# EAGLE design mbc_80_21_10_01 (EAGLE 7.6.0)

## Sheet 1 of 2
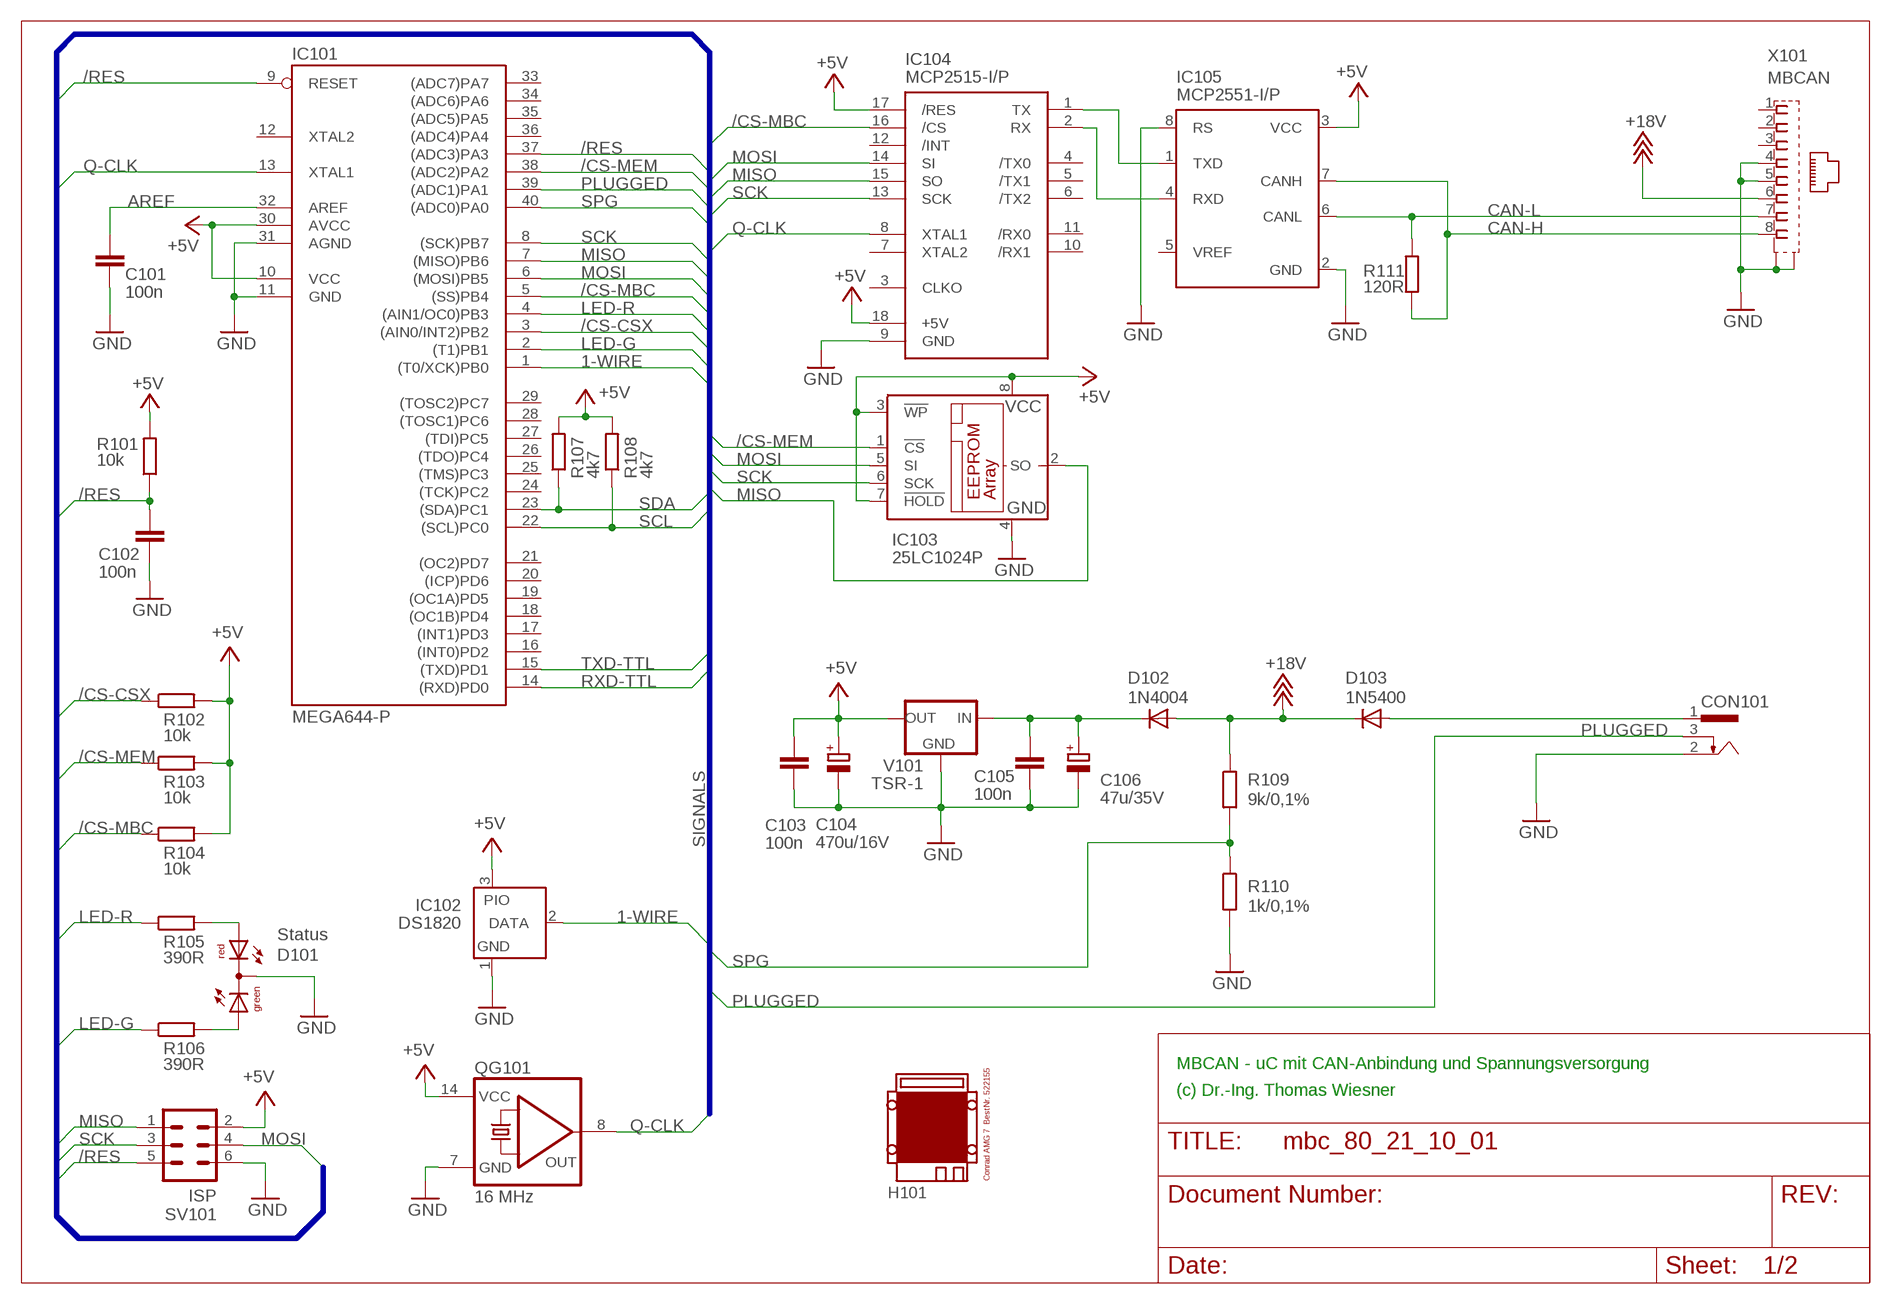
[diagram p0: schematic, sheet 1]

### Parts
C101  100n  C-EU025-025X050  [C025-025X050]
C102  100n  C-EU025-025X050  [C025-025X050]
C103  100n  C-EU025-025X050  [C025-025X050]
C104  470u/16V  CPOL-EUE3.5-8  [E3,5-8]
C105  100n  C-EU025-025X050  [C025-025X050]
C106  47u/35V  CPOL-EUE2.5-7  [E2,5-7]
CON101  POWER-JACK  [POWER-JACK]
D101  Status  DUOLED5MM  [DUOLED5MM]
D102  1N4004  [DO41-10]
D103  1N5400  [DO201-15]
H101  MODULGEHÄUSE-AMG-7  [MODULGEHÄUSE-AMG-7]
IC101  MEGA644-P  MEGA323-P  [DIL40]
IC102  DS1820  DS2405  [TO92-]
IC103  25LC1024P  25LC040P  [DIL8]
IC104  MCP2515-I/P  MCP2510-I/P  [DIL18]
IC105  MCP2551-I/P  PCA82C250  [DIL08]
QG101  16 MHz  QG5860  [DIL14S]
R101  10k  R-EU_0207/10  [0207/10]
R102  10k  R-EU_0207/10  [0207/10]
R103  10k  R-EU_0207/10  [0207/10]
R104  10k  R-EU_0207/10  [0207/10]
R105  390R  R-EU_0207/10  [0207/10]
R106  390R  R-EU_0207/10  [0207/10]
R107  4k7  R-EU_0207/10  [0207/10]
R108  4k7  R-EU_0207/10  [0207/10]
R109  9k/0,1%  R-EU_0207/10  [0207/10]
R110  1k/0,1%  R-EU_0207/10  [0207/10]
R111  120R  R-EU_0207/10  [0207/10]
SV101  ISP  ML6  [ML6]
V101  TSR-1  [TRACO-TSR-1]
X101  MBCAN  0446200002  [0446200002]

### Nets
1-WIRE: IC101.1((T0/XCK)PB0) IC102.2(DATA)
+5V: C103.1 C104.+ IC101.10(VCC) IC101.30(AVCC) IC102.3(PIO) IC103.3(!WP) IC103.7(!HOLD) IC103.8(VCC) IC104.17(/RES) IC104.18(+5V) IC105.3(VCC) QG101.14(VCC) R101.2 R102.2 R103.2 R104.2 R107.2 R108.2 SV101.2 V101.OUT ; also sheet 2
+18V: D102.A D103.C R109.1 X101.6
/CS-CSX: IC101.3((AIN0/INT2)PB2) R102.1 ; also sheet 2
/CS-MBC: IC101.5((SS)PB4) IC104.16(/CS) R104.1
/CS-MEM: IC101.38((ADC2)PA2) IC103.1(!CS) R103.1
/RES: C102.1 IC101.9(RESET) IC101.37((ADC3)PA3) R101.1 SV101.5
AREF: C101.1 IC101.32(AREF)
CAN-H: IC105.7(CANH) R111.1 X101.8
CAN-L: IC105.6(CANL) R111.2 X101.7
GND: C101.2 C102.2 C103.2 C104.- C105.2 C106.- CON101.2 D101.K(C) IC101.11(GND) IC101.31(AGND) IC102.1(GND) IC103.4(GND) IC104.9(GND) IC105.2(GND) IC105.8(RS) QG101.7(GND) R110.2 SV101.6 V101.GND X101.4 X101.5 X101.S@1(S1) X101.S@2(S2) ; also sheet 2
LED-G: IC101.2((T1)PB1) R106.1
LED-R: IC101.4((AIN1/OC0)PB3) R105.1
MISO: IC101.7((MISO)PB6) IC103.2(SO) IC104.15(SO) SV101.1 ; also sheet 2
MOSI: IC101.6((MOSI)PB5) IC103.5(SI) IC104.14(SI) SV101.4 ; also sheet 2
N$1: IC104.1(TX) IC105.1(TXD)
N$2: IC104.2(RX) IC105.4(RXD)
N$6: C105.1 C106.+ D102.C V101.IN
N$9: D101.AR R105.2
N$13: D101.AG R106.2
PLUGGED: CON101.3 IC101.39((ADC1)PA1)
Q-CLK: IC101.13(XTAL1) IC104.8(XTAL1) QG101.8(OUT) ; also sheet 2
RXD-TTL: IC101.14((RXD)PD0) ; also sheet 2
SCK: IC101.8((SCK)PB7) IC103.6(SCK) IC104.13(SCK) SV101.3 ; also sheet 2
SCL: IC101.22((SCL)PC0) R108.1 ; also sheet 2
SDA: IC101.23((SDA)PC1) R107.1 ; also sheet 2
SPG: IC101.40((ADC0)PA0) R109.2 R110.1
TXD-TTL: IC101.15((TXD)PD1) ; also sheet 2
V-NETZTEIL: CON101.1 D103.A
Unconnected: IC101.12(XTAL2) IC101.16((INT0)PD2) IC101.17((INT1)PD3) IC101.18((OC1B)PD4) IC101.19((OC1A)PD5) IC101.20((ICP)PD6) IC101.21((OC2)PD7) IC101.24((TCK)PC2) IC101.25((TMS)PC3) IC101.26((TDO)PC4) IC101.27((TDI)PC5) IC101.28((TOSC1)PC6) IC101.29((TOSC2)PC7) IC101.33((ADC7)PA7) IC101.34((ADC6)PA6) IC101.35((ADC5)PA5) IC101.36((ADC4)PA4) IC104.3(CLKO) IC104.4(/TX0) IC104.5(/TX1) IC104.6(/TX2) IC104.7(XTAL2) IC104.10(/RX1) IC104.11(/RX0) IC104.12(/INT) IC105.5(VREF) X101.1 X101.2 X101.3

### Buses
SIGNALS

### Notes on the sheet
- MBCAN - uC mit CAN-Anbindung und Spannungsversorgung
- (c) Dr.-Ing. Thomas Wiesner

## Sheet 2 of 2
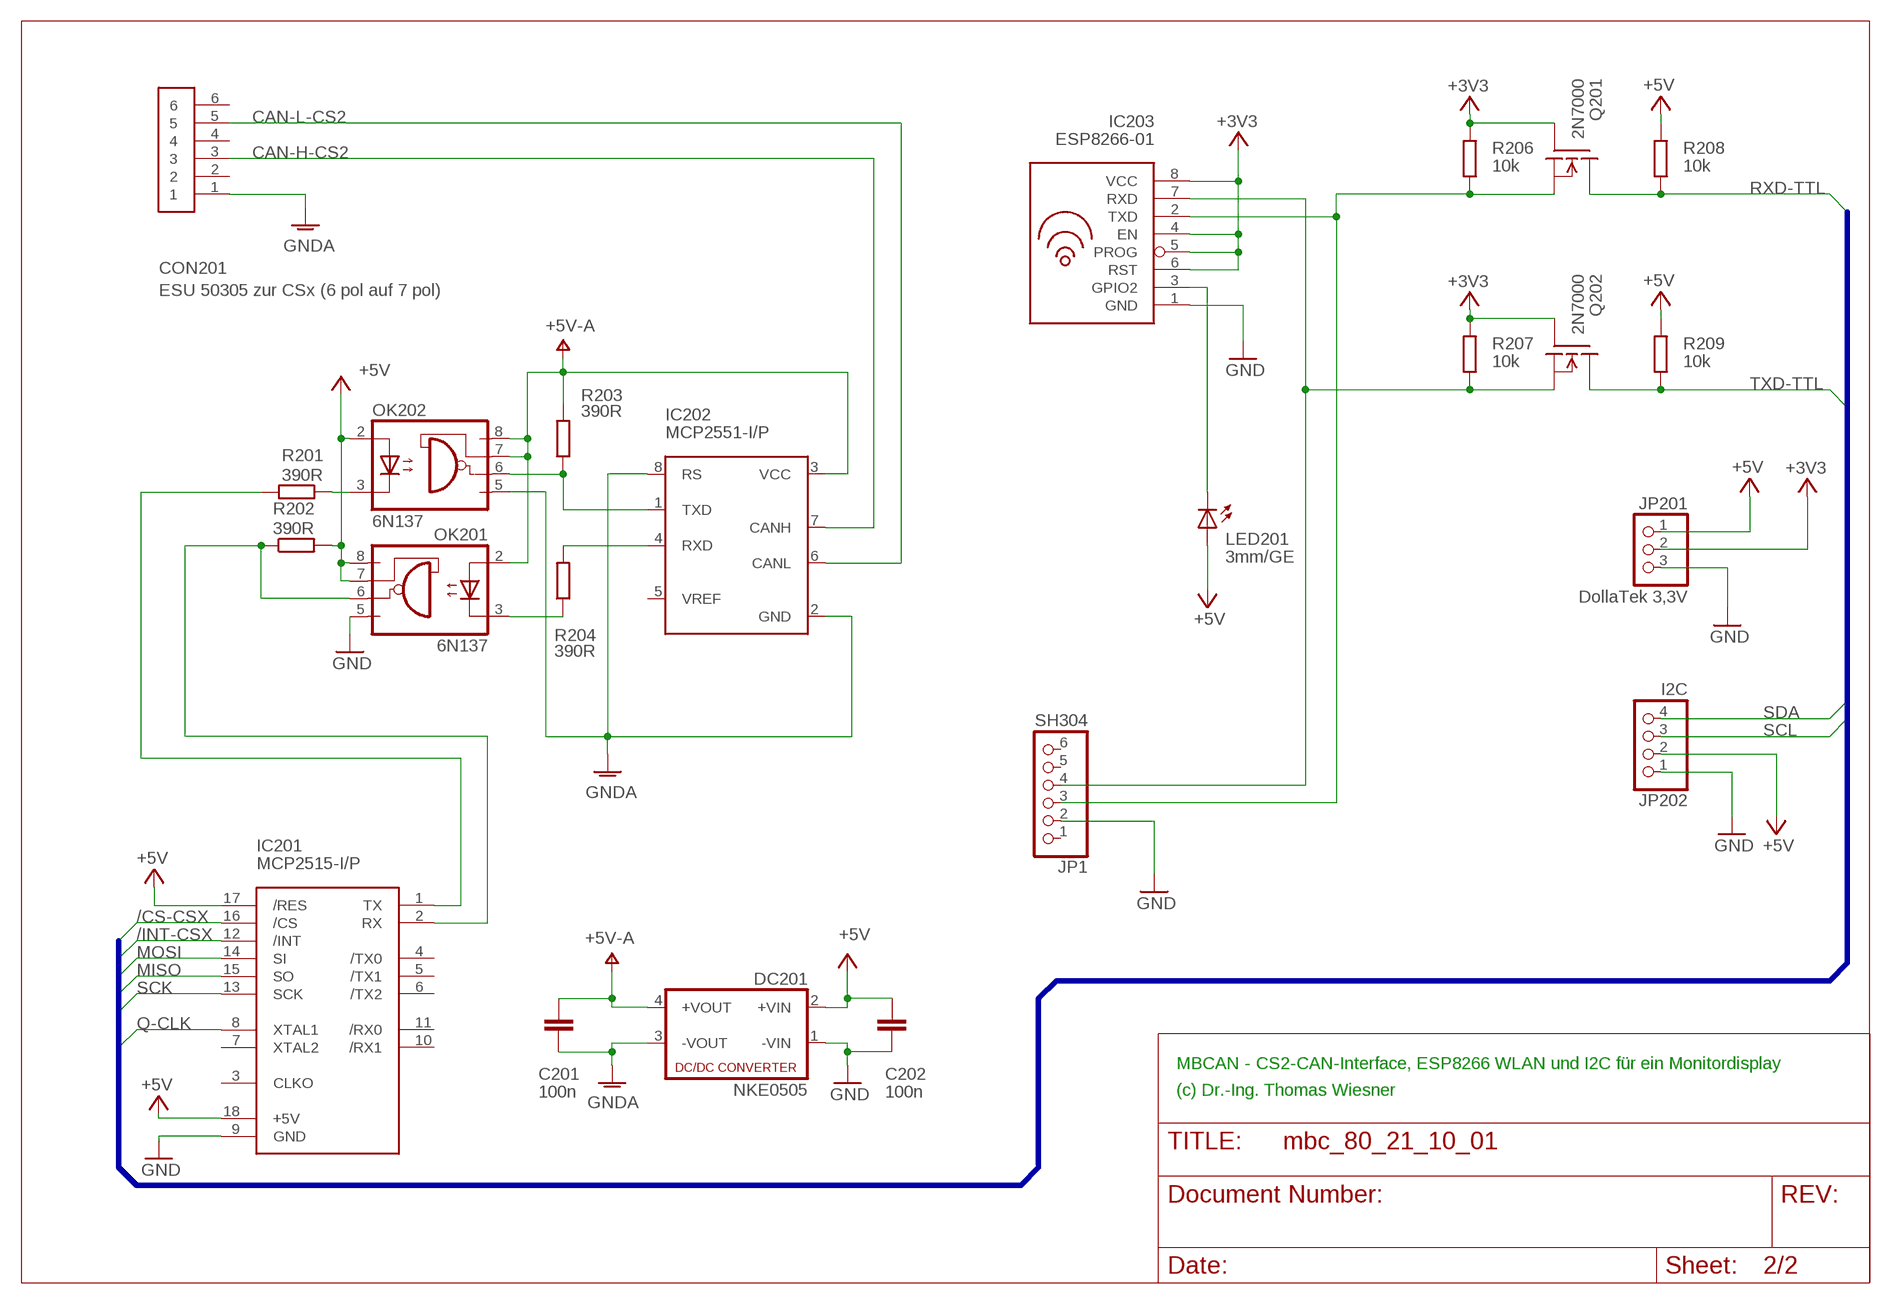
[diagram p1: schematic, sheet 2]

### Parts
C201  100n  C-EU025-025X050  [C025-025X050]
C202  100n  C-EU025-025X050  [C025-025X050]
CON201  ESU 50305 zur CSx (6 pol auf 7 pol)  TM-0508-A6  [MINI-DIN-6-POL]
DC201  NKE0505  NME  [NME]
IC201  MCP2515-I/P  MCP2510-I/P  [DIL18]
IC202  MCP2551-I/P  PCA82C250  [DIL08]
IC203  ESP8266-01  [ESP8266-01]
JP1  SH304  PINHD-1X6  [1X06]
JP201  DollaTek 3,3V  PINHD-1X3  [1X03]
JP202  I2C  PINHD-1X4  [1X04]
LED201  3mm/GE  LED3MM  [LED3MM]
OK201  6N137  [DIL08]
OK202  6N137  [DIL08]
Q201  2N7000  TN0602N3  [TO-92]
Q202  2N7000  TN0602N3  [TO-92]
R201  390R  R-EU_0207/10  [0207/10]
R202  390R  R-EU_0207/10  [0207/10]
R203  390R  R-EU_0207/10  [0207/10]
R204  390R  R-EU_0207/10  [0207/10]
R206  10k  R-EU_0207/10  [0207/10]
R207  10k  R-EU_0207/10  [0207/10]
R208  10k  R-EU_0207/10  [0207/10]
R209  10k  R-EU_0207/10  [0207/10]

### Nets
+3V3: IC203.4(EN) IC203.5(PROG) IC203.6(RST) IC203.8(VCC) JP201.2 Q201.2(G) Q202.2(G) R206.2 R207.2
+5V: C202.1 DC201.2(+VIN) IC201.17(/RES) IC201.18(+5V) JP201.1 JP202.2 LED201.A OK201.7(VE) OK201.8(VCC) OK202.2(A) R202.2 R208.2 R209.2 ; also sheet 1
+5V-A: C201.1 DC201.4(+VOUT) IC202.3(VCC) OK201.2(A) OK202.7(VE) OK202.8(VCC) R203.2
/CS-CSX: IC201.16(/CS) ; also sheet 1
/INT-CSX: IC201.12(/INT)
CAN-H-CS2: CON201.3 IC202.7(CANH)
CAN-L-CS2: CON201.5 IC202.6(CANL)
GND: C202.2 DC201.1(-VIN) IC201.9(GND) IC203.1(GND) JP1.2 JP201.3 JP202.1 OK201.5(GND) ; also sheet 1
GNDA: C201.2 CON201.1 DC201.3(-VOUT) IC202.2(GND) IC202.8(RS) OK202.5(GND)
MISO: IC201.15(SO) ; also sheet 1
MOSI: IC201.14(SI) ; also sheet 1
N$3: IC203.3(GPIO2) LED201.K(C)
N$5: IC203.2(TXD) JP1.3 Q201.1(S) R206.1
N$8: IC203.7(RXD) JP1.4 Q202.1(S) R207.1
N$10: IC201.1(TX) R201.2
N$40: IC202.1(TXD) OK202.6(VO) R203.1
N$43: OK201.3(C) R204.1
N$44: IC202.4(RXD) R204.2
N$46: OK202.3(C) R201.1
N$48: IC201.2(RX) OK201.6(VO) R202.1
Q-CLK: IC201.8(XTAL1) ; also sheet 1
RXD-TTL: Q201.3(D) R208.1 ; also sheet 1
SCK: IC201.13(SCK) ; also sheet 1
SCL: JP202.3 ; also sheet 1
SDA: JP202.4 ; also sheet 1
TXD-TTL: Q202.3(D) R209.1 ; also sheet 1
Unconnected: CON201.2 CON201.4 CON201.6 IC201.3(CLKO) IC201.4(/TX0) IC201.5(/TX1) IC201.6(/TX2) IC201.7(XTAL2) IC201.10(/RX1) IC201.11(/RX0) IC202.5(VREF) JP1.1 JP1.5 JP1.6

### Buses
SIGNALS

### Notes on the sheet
- MBCAN - CS2-CAN-Interface, ESP8266 WLAN und I2C für ein Monitordisplay
- (c) Dr.-Ing. Thomas Wiesner

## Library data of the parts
C101-C103 C105 C201 C202 = rcl:C-EU: CAPACITOR, European symbol
C104 C106 = rcl:CPOL-EU: POLARIZED CAPACITOR, European symbol
CON101 = mbc:POWER-JACK
CON201 = mbc:TM-0508-A6: MINI-DIN 6-pol Printbuchse Reichelt Bestellnummer EB-DIO M06
D101 = led:DUOLED5MM: DUO LED 2 colors, 5 mm, round
D102 = diode:1N4004: DIODE
D103 = diode:1N5400: DIODE
DC201 = dc-dc-converter:NME: DC-DC CONVERTER; MF: C & D TECHNOLOGIES, INC; MPN: NME1205D; OC_FARNELL: 1021466; OC_NEWARK: 98B8198
H101 = mbc:MODULGEHÄUSE-AMG-7: Gehäuse
IC101 = atmel:MEGA323-P: MICROCONTROLLER 32 Kbytes FLASH 2 Kbytes SRAM 1 Kbytes EEPROM USART 8-channel 10 bit ADC Source: avr.lbr; OC_FARNELL: unknown; OC_NEWARK: unknown
IC102 = maxim:DS2405: Addressable Switch DALLAS Semiconductor; MF: DALLAS SEMICONDUCTOR; MPN: DS2405; OC_FARNELL: 1188025; OC_NEWARK: 06F4645
IC103 = microchip:25*: Serial EEPROM 4K/ 8K , SPI bus; MF: MICROCHIP; MPN: 25LC040/P; OC_FARNELL: 9758100; OC_NEWARK: 96K4091
IC104 IC201 = mbc:MCP2510: BASIC-CAN 2.0a Controller Stand-alone CAN controller von Microchip
IC105 IC202 = micro-philips:PCA82C250: CAN CONTROLLER INTERFACE; OC_FARNELL: 3692358; OC_NEWARK: unknown
IC203 = mbc:ESP8266-01
JP1 = pinhead:PINHD-1X6: PIN HEADER
JP201 = pinhead:PINHD-1X3: PIN HEADER
JP202 = pinhead:PINHD-1X4: PIN HEADER
LED201 = led:LED: LED
OK201 OK202 = optocoupler:6N137: MOTOROLA OPTO COUPLER; MPN: 6N137; OC_FARNELL: 1328376; OC_NEWARK: 52M1895
Q201 Q202 = transistor-fet:TN0602N3: N-Channel Enhancement MOSFET 20V; 4A; 0,75Ohm
QG101 = crystal:QG5860: CRYSTAL RESONATOR; OC_FARNELL: unknown; OC_NEWARK: unknown
R101-R111 R201-R204 R206-R209 = resistor:R-EU_: RESISTOR, European symbol
SV101 = con-ml:ML6: HARTING; OC_FARNELL: unknown; OC_NEWARK: unknown
V101 = mbc:TSR-1: Spannungsregler Hersteller: TRACO Typ: TSR-1 5V: TSR 1-2450 Spg: 5V Strom: 1A Reichelt TSR 1-2450
X101 = mbc:0446200002: RJ-45 INVERTED MODULAR JACK ASSEMBLY WITH RJ-11 KEEPOUT FEATURE Source: Data sheet MOLEX 0446200002 BUCHSE, RJ45, GESCHIRMT Source: Farnell; MF: MOLEX; MPN: 0446200002; OC_FARNELL: 9251910

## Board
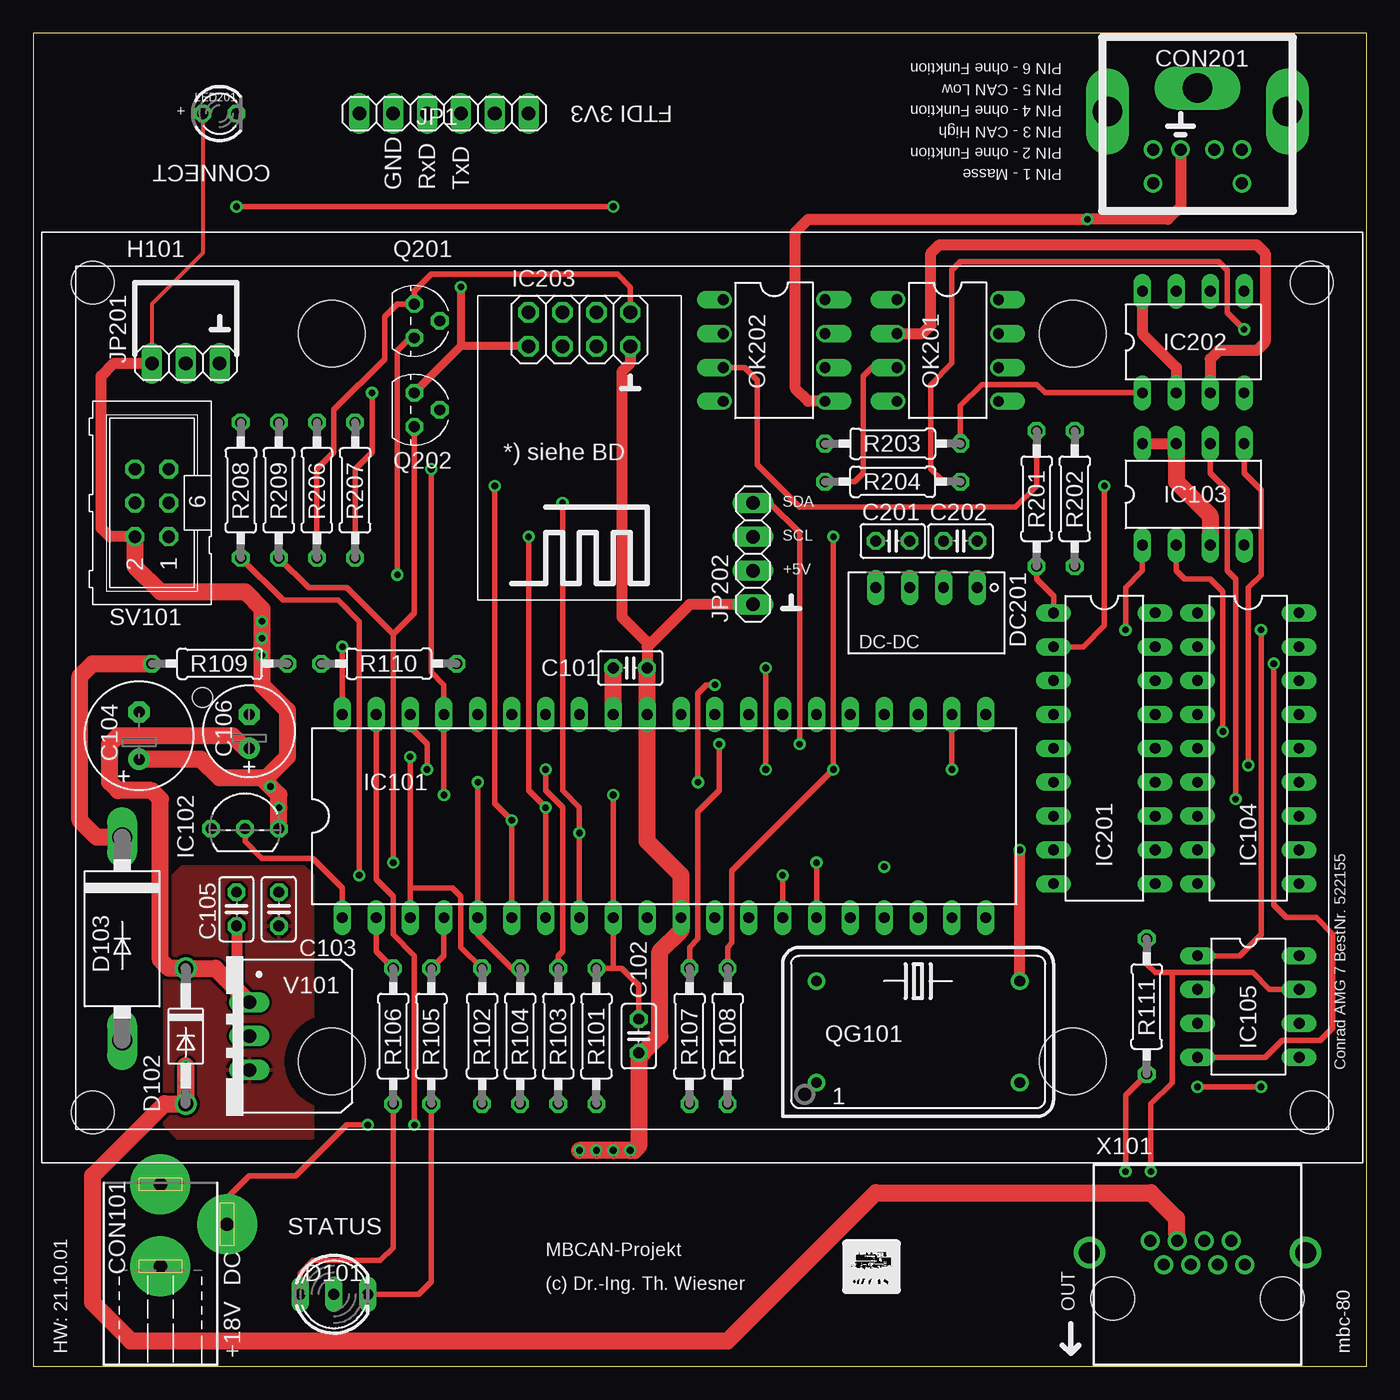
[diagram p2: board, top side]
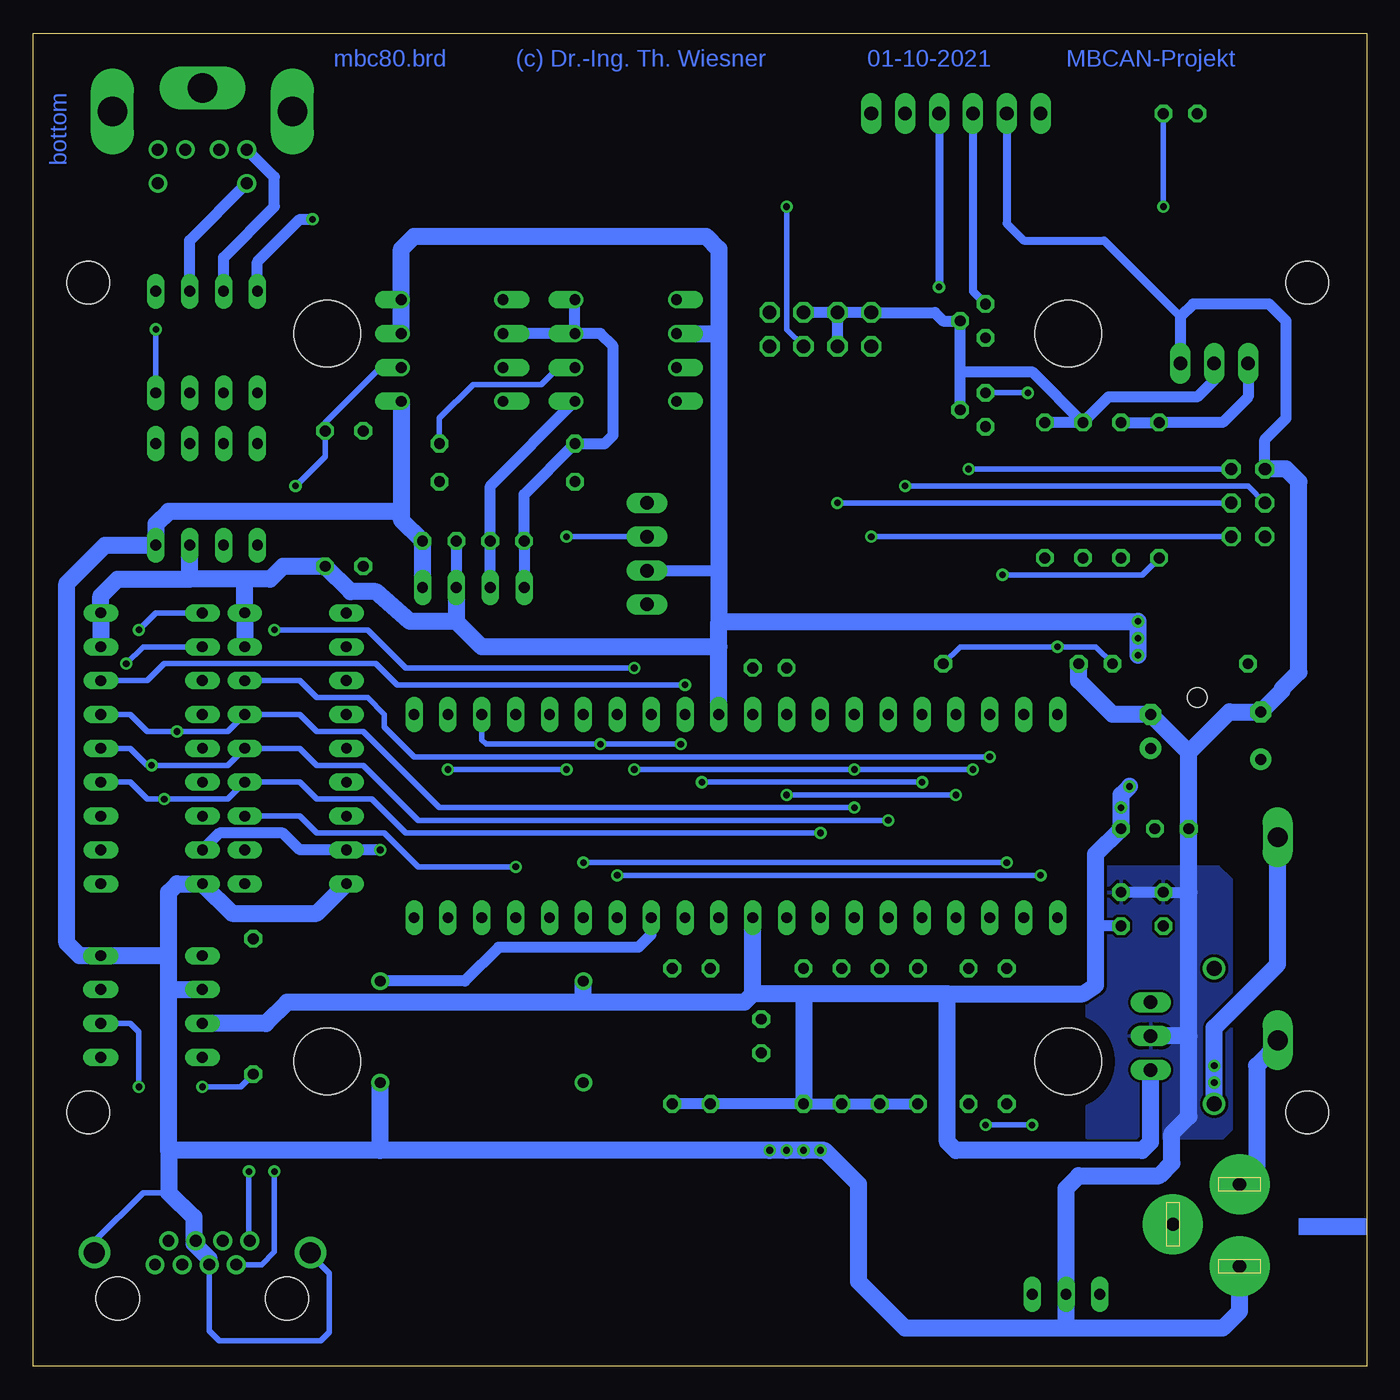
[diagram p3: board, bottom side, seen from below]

Size 99.99 x 100 mm. Coordinates in mm from the lower left corner, seen from the top.
Outline: 0,0 99.99,0 99.99,100 0,100 0,0
Copper layers (1*16): Top 0.035mm / dielectric 1.5mm / Bottom 0.035mm
Design rules "default *": minimum track width 10mil, minimum drill 0.5mm, track to track 8mil, track to pad 8mil, pad to pad 8mil, via to via 8mil, smd to smd 8mil, copper to edge 40mil, drill to drill 8mil, minimum pad ring 10mil, minimum via ring 8mil, stop-mask expansion 4mil, vias tented up to drill 0mil, thermal gap 10mil

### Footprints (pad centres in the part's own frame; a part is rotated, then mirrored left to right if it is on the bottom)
C025-025X050 = drill 0.813 octagon: 1 -1.27,0; 2 1.27,0
E3,5-8 = drill 0.813 pad 1.6: + -1.778,0 | drill 0.813 pad 1.6 octagon: - 1.778,0
E2,5-7 = drill 0.813 pad 1.6: + -1.27,0 | drill 0.813 pad 1.6 octagon: - 1.27,0
POWER-JACK = drill 1 pad 4.5: 1 0,6.03; 2 0,-0.12; 3 5,3.03
MINI-DIN-6-POL = drill 0.9: 1 -1.27,-4.604; 2 1.27,-4.604; 3 -3.334,-4.604; 4 3.334,-4.604; 5 -3.334,-7.144; 6 3.334,-7.144 | drill 2.2 pad 2.54 long: A1 0,0.01; A2 -6.75,-1.746; A3 6.75,-1.746
DUOLED5MM = drill 0.813 long: AG -2.54,0; AR 2.54,0; K 0,0
DO41-10 = drill 1.118: A 5.08,0; C -5.08,0
DO201-15 = drill 1.499 long: A 7.62,0; C -7.62,0
NME = drill 0.813 long: 1 0,3.81; 2 0,1.27; 3 0,-1.27; 4 0,-3.81
MODULGEHÄUSE-AMG-7 = hole 3.2: -45.72,-31.115; -45.72,31.115; 45.72,31.115; 45.72,-31.115 | hole 5: -27.781,-27.305; 27.781,-27.305; -27.781,27.305; 27.781,27.305 | hole 1.5: -37.465,0
DIL40 = drill 0.813 long: 1 -24.13,-7.62; 2 -21.59,-7.62; 3 -19.05,-7.62; 4 -16.51,-7.62; 5 -13.97,-7.62; 6 -11.43,-7.62; 7 -8.89,-7.62; 8 -6.35,-7.62; 9 -3.81,-7.62; 10 -1.27,-7.62; 11 1.27,-7.62; 12 3.81,-7.62; 13 6.35,-7.62; 14 8.89,-7.62; 15 11.43,-7.62; 16 13.97,-7.62; 17 16.51,-7.62; 18 19.05,-7.62; 19 21.59,-7.62; 20 24.13,-7.62; 21 24.13,7.62; 22 21.59,7.62; 23 19.05,7.62; 24 16.51,7.62; 25 13.97,7.62; 26 11.43,7.62; 27 8.89,7.62; 28 6.35,7.62; 29 3.81,7.62; 30 1.27,7.62; 31 -1.27,7.62; 32 -3.81,7.62; 33 -6.35,7.62; 34 -8.89,7.62; 35 -11.43,7.62; 36 -13.97,7.62; 37 -16.51,7.62; 38 -19.05,7.62; 39 -21.59,7.62; 40 -24.13,7.62
TO92- = drill 0.813 octagon: 1 -2.54,0; 2 0,0; 3 2.54,0
DIL8 = drill 0.813 long: 1 -3.81,-3.81; 2 -1.27,-3.81; 3 1.27,-3.81; 4 3.81,-3.81; 5 3.81,3.81; 6 1.27,3.81; 7 -1.27,3.81; 8 -3.81,3.81
DIL18 = drill 0.813 long: 1 -10.16,-3.81; 2 -7.62,-3.81; 3 -5.08,-3.81; 4 -2.54,-3.81 | drill 0.8 long: 5 0,-3.81; 6 2.54,-3.81; 7 5.08,-3.81; 8 7.62,-3.81; 9 10.16,-3.81; 10 10.16,3.81; 11 7.62,3.81; 12 5.08,3.81; 13 2.54,3.81; 14 0,3.81; 15 -2.54,3.81; 16 -5.08,3.81; 17 -7.62,3.81; 18 -10.16,3.81
DIL08 = drill 0.813 long: 1 -3.81,-3.81; 2 -1.27,-3.81; 3 1.27,-3.81; 4 3.81,-3.81; 5 3.81,3.81; 6 1.27,3.81; 7 -1.27,3.81; 8 -3.81,3.81
ESP8266-01 = drill 1.016 octagon: 1 3.81,-1.27; 2 3.81,1.27; 3 1.27,-1.27; 4 1.27,1.27; 5 -1.27,-1.27; 6 -1.27,1.27; 7 -3.81,-1.27; 8 -3.81,1.27
1X06 = drill 1.016 long: 1 -6.35,0; 2 -3.81,0; 3 -1.27,0; 4 1.27,0; 5 3.81,0; 6 6.35,0
1X03 = drill 1.016 long: 1 -2.54,0; 2 0,0; 3 2.54,0
1X04 = drill 1.016 long: 1 -3.81,0; 2 -1.27,0; 3 1.27,0; 4 3.81,0
LED3MM = drill 0.813 octagon: A -1.27,0; K 1.27,0
DIL08' = drill 0.813 offset: 1 -3.81,-3.81; 2 -1.27,-3.81; 3 1.27,-3.81; 4 3.81,-3.81; 5 3.81,3.81; 6 1.27,3.81; 7 -1.27,3.81; 8 -3.81,3.81
TO-92 = drill 0.813 octagon: 1 -1.27,0; 2 0,1.905; 3 1.27,0
DIL14S = drill 0.813: 1 -7.62,-3.81; 7 7.62,-3.81; 8 7.62,3.81; 14 -7.62,3.81
0207/10 = drill 0.813 octagon: 1 -5.08,0; 2 5.08,0
ML6 = drill 0.914 octagon: 1 -2.54,-1.27; 2 -2.54,1.27; 3 0,-1.27; 4 0,1.27; 5 2.54,-1.27; 6 2.54,1.27
TRACO-TSR-1 = drill 1.016 long: GND 0,2.54; IN -2.54,2.54; OUT 2.54,2.54
0446200002 = drill 0.889 pad 1.422: 1 3.556,2.54; 2 2.54,4.318; 3 1.524,2.54; 4 0.508,4.318; 5 -0.508,2.54; 6 -1.524,4.318; 7 -2.54,2.54; 8 -3.556,4.318 | drill 1.575 pad 2.286: S@1 -8.103,3.429; S@2 8.103,3.429 | hole 3.251: 6.35,0; -6.35,0

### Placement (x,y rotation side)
C101  44.77,52.39 0 top
C102  45.4,24.77 270 top
C103  18.41,34.29 90 top
C104  7.94,47.31 90 top
C105  15.24,34.29 90 top
C106  16.19,47.62 90 top
C201  64.45,61.91 0 top
C202  69.53,61.91 0 top
CON101  9.53,7.62 0 top
CON201  87.31,95.89 0 top
D101  22.54,5.4 0 top
D102  11.43,24.77 270 top
D103  6.67,32.07 270 top
DC201  66.99,58.42 270 top
H101  50.16,50.16 0 top
IC101  47.31,41.27 0 top
IC102  15.88,40.32 0 top
IC103  87,65.41 0 top
IC104  91.12,46.35 270 top
IC105  91.12,26.99 270 top
IC201  80.33,46.35 270 top
IC202  87,76.83 0 top
IC203  40.96,77.79 0 top
JP1  30.8,93.98 0 top
JP201  11.43,75.25 0 top
JP202  53.98,60.96 90 top
LED201  13.97,93.98 0 top
OK201  6N137  [DIL08']  68.58,76.2 270 top
OK202  6N137  [DIL08']  55.56,76.2 270 top
Q201  28.57,78.42 270 top
Q202  28.57,71.75 270 top
QG101  66.36,25.08 0 top
R101  42.23,24.77 270 top
R102  33.66,24.77 270 top
R103  39.37,24.77 270 top
R104  36.51,24.77 270 top
R105  29.84,24.77 270 top
R106  26.99,24.77 270 top
R107  49.21,24.77 270 top
R108  52.07,24.77 270 top
R109  13.97,52.7 0 top
R110  26.67,52.7 180 top
R111  83.5,26.99 270 top
R201  75.25,65.09 270 top
R202  78.11,65.09 270 top
R203  64.45,69.22 180 top
R204  64.45,66.36 0 top
R206  21.27,65.72 90 top
R207  24.13,65.72 90 top
R208  15.56,65.72 90 top
R209  18.41,65.72 90 top
SV101  8.89,64.77 90 top
V101  13.65,24.77 270 top
X101  87.31,5.08 0 top

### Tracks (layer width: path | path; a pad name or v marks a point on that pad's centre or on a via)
1-WIRE
  Top 0.406: IC102.2 15.88,39.37 17.14,38.1 20.95,38.1 23.18,35.88 IC101.1
+3V3
  Bottom 0.813: 30.48,74.61 Q201.2 31.75,78.42 32.38,79.06 IC203.8 IC203.6 | R206.2 R207.2 | JP201.2 11.43,73.98 12.7,72.71 19.37,72.71 R206.2 | Q202.2 30.48,74.61 | 30.48,74.61 25.08,74.61 R206.2 | IC203.6 IC203.4 | IC203.6 IC203.5
+5V  (via drill 0.5)
  Top 0.305: LED201.A 12.7,83.5 8.89,79.69 JP201.1
  Top 0.813: IC103.8 IC103.7 | SV101.2 5.71,62.23 5.08,62.87 5.08,74.3 6.03,75.25 JP201.1
  Top 1.27: C104.+ 12.57,45.53 13.97,44.13 17.14,44.13 | IC102.3 v18.41,41.91 18.41,42.86 v17.78,43.5 17.14,44.13 | SV101.2 7.62,60.01 9.53,58.1 15.88,58.1 17.14,56.83 v17.14,55.88 v17.14,54.61 v17.14,53.34 17.14,51.12 19.05,49.21 19.05,45.72 17.46,44.13 17.14,44.13 | IC103.7 85.72,66.36 88.27,63.82 IC103.3
  Bottom 0.813: R209.2 R208.2 10.79,70.8 8.89,72.71 JP201.1 | C202.1 DC201.2 | C103.1 20.32,33.02 | JP202.2 48.58,59.69 | R108.2 R107.2 R101.2 R103.2 R104.2 R102.2
  Bottom 1.016: 88.27,59.69 88.42,59.21 88.58,59.05
  Bottom 1.27: IC104.17 IC104.18 94.93,57.78 93.66,59.05 88.58,59.05 | IC201.17 IC201.18 84.14,59.05 | 46.04,27.94 IC101.10 | 58.74,27.3 46.67,27.3 46.04,27.94 | 58.74,27.3 QG101.14 | 42.23,27.94 R101.2 | 31.43,27.94 21.27,27.94 20.32,28.57 20.32,33.02 20.32,38.42 IC102.3 v18.41,41.91 18.41,42.86 v17.78,43.5 | 31.43,27.94 42.23,27.94 | 42.23,27.94 46.04,27.94 | IC105.3 82.55,25.72 80.96,27.3 58.74,27.3 | V101.OUT 16.19,16.83 16.83,16.19 30.8,16.19 31.43,16.83 31.43,27.94 | IC101.30 48.58,53.98 | 48.58,53.98 48.58,55.88 | 48.58,55.88 v17.14,55.88 v17.14,54.61 v17.14,53.34 | 84.14,59.05 88.27,59.05 88.42,59.21 | 88.27,59.69 IC103.3 | OK201.8 OK201.7 72.39,83.82 71.44,84.77 49.53,84.77 48.58,83.82 48.58,77.47 | 48.58,77.47 48.58,59.69 48.58,55.88 | OK202.2 48.58,77.47 | 48.58,53.98 66.36,53.98 68.26,55.88 | DC201.2 68.26,55.88 | 68.26,55.88 71.75,55.88 74.3,58.1 76.2,58.1 R202.2 81.28,60.01 82.23,59.05 84.14,59.05
  pour Top: 11.11,37.47 20.32,37.47 20.95,36.83 20.95,17.14 10.79,17.14 9.84,18.1 9.84,36.2
+5V-A
  Top 0.813: OK201.2 66.67,77.47 67.31,78.11 67.31,83.5 67.94,84.14 91.76,84.14 92.39,83.5 92.39,76.83 91.76,76.2 88.9,76.2 88.27,75.56 IC202.3
  Bottom 0.813: DC201.4 C201.1 63.18,65.41 R203.2 57.15,69.22 56.52,69.85 56.52,76.52 57.47,77.47 OK202.7 | OK202.7 OK202.8 | OK202.7 OK201.2
+18V  (via drill 0.5)
  Top 1.27: R109.1 4.45,52.7 3.49,51.75 3.49,40.96 4.76,39.69 D103.C | D102.A 9.84,19.68 4.45,14.29 4.45,4.76 7.3,1.91 52.07,1.91 63.18,13.02 83.82,13.02 85.72,11.11 85.72,10.1 X101.6 | D102.A v11.43,21.27 v11.43,22.54 D102.A
  Bottom 1.27: D103.C 6.67,30.16 11.43,25.4 v11.43,21.27 D102.A
/CS-CSX  (via drill 0.5)
  Top 0.406: IC101.3 28.26,35.88 | 28.26,35.88 v28.26,45.72 | 28.26,35.88 31.43,35.88 32.07,35.24 32.07,31.43 R102.1
  Bottom 0.406: IC201.16 80.01,51.44 78.74,50.16 74.93,50.16 73.66,48.9 73.66,47.94 71.44,45.72 v28.26,45.72
/CS-MBC  (via drill 0.5)
  Top 0.406: v33.34,43.81 IC101.5 33.34,32.38 35.88,29.84 R104.1 | v49.85,43.81 49.85,50.48 50.48,51.12 v51.12,51.12
  Bottom 0.406: IC104.16 91.44,51.44 90.17,52.7 74.3,52.7 72.71,51.12 v51.12,51.12 | v49.85,43.81 v33.34,43.81
/CS-MEM  (via drill 0.5)
  Top 0.406: v29.53,44.77 29.53,46.67 28.26,47.94 IC101.38 | v81.92,55.24 81.92,58.42 83.19,59.69 IC103.1 | v54.93,44.77 v54.93,52.39 | R103.1 39.37,30.8 39.69,31.11 39.69,41.91 38.42,43.18 v38.42,44.77
  Bottom 0.406: v54.93,44.77 v38.42,44.77 v29.53,44.77 | v81.92,55.24 74.93,55.24 72.07,52.39 v54.93,52.39
/INT-CSX  (via drill 0.5)
  Bottom 0.406: IC201.12 80.01,41.27 78.74,40.01 73.66,40.01 71.12,37.47 v63.82,37.47
/RES  (via drill 0.5)
  Top 0.406: 43.5,29.84 IC101.9 v43.5,42.86 | R101.1 43.5,29.84 | 43.5,29.84 44.13,29.84 45.4,28.57 C102.1 | v29.84,67.31 29.84,52.07 30.8,51.12 IC101.37 v30.8,42.86
  Bottom 0.406: SV101.5 v29.84,67.31 | v30.8,42.86 v43.5,42.86
AREF
  Top 1.27: IC101.32 C101.1
CAN-H  (via drill 0.5)
  Top 0.406: v83.82,14.61 83.82,19.68 85.41,21.27 85.41,29.53 | 85.41,29.53 91.44,29.53 92.71,28.26 IC105.7 | R111.1 83.5,30.16 84.14,29.53 85.41,29.53
  Bottom 0.406: X101.8 83.82,9.4 v83.82,14.61
CAN-H-CS2
  Bottom 0.813: IC202.7 85.72,83.19 81.92,87 81.92,89.22 CON201.3
CAN-L  (via drill 0.5)
  Top 0.406: v81.92,14.61 81.92,20.32 R111.2 | v92.08,20.95 v87.31,20.95
  Bottom 0.406: X101.7 82.87,7.62 81.92,8.57 v81.92,14.61 | IC105.6 92.71,25.72 92.08,25.08 v92.08,20.95 | v87.31,20.95 84.45,20.95 R111.2
CAN-L-CS2
  Bottom 0.813: IC202.6 88.27,84.45 CON201.5
GND  (via drill 0.5)
  Top 0.813: IC203.1 44.77,75.25 44.13,74.61 44.13,56.2 46.04,54.29 46.04,53.98 | 46.04,53.98 C101.2 | JP202.1 49.21,57.15 46.04,53.98
  Top 1.27: C101.2 IC101.31 46.04,39.37 48.58,36.83 IC101.11 48.58,32.7 46.99,31.11 46.99,24.77 45.72,23.5 C102.2 45.4,16.51 45.09,16.19 v44.77,16.19 v43.5,16.19 v42.23,16.19 v40.96,16.19
  Bottom 0.406: X101.S@2 95.42,9.36 91.76,13.02 89.85,13.02 | X101.5 86.81,2.67 86.04,1.91 78.42,1.91 77.79,2.54 77.79,6.99 79.06,8.26 79.15,8.26 X101.S@1
  Bottom 0.61: 35.56,3.49 35.56,3.81 | JP1.2 26.99,85.72 25.72,84.45 19.68,84.45 13.97,78.74
  Bottom 0.813: IC105.8 95.25,30.8 | SV101.6 7.62,69.53 6.03,71.12 6.03,78.42 7.3,79.69 13.02,79.69 13.97,78.74 JP201.3 | 13.34,35.56 C105.2 C103.2
  Bottom 1.27: 22.54,2.86 10.79,2.86 9.53,4.13 CON101.2 | 22.54,2.86 D101.K 22.54,13.34 21.59,14.29 15.56,14.29 14.61,15.24 14.61,17.46 13.34,18.73 13.34,24.77 | 22.54,2.86 34.61,2.86 35.56,3.81 38.1,6.35 38.1,13.65 40.64,16.19 v40.96,16.19 v42.23,16.19 v43.5,16.19 v44.77,16.19 73.98,16.19 | 73.98,16.19 89.85,16.19 | 73.98,16.19 QG101.7 | 13.34,24.77 13.34,35.56 IC102.1 13.34,46.04 | 13.34,46.04 C106.- 19.05,48.9 21.59,51.44 R110.2 | 13.34,46.04 10.29,49.09 C104.- 6.35,50.67 6.35,50.8 5.08,52.07 5.08,66.36 6.03,67.31 SV101.6 | 89.85,16.19 89.85,28.26 | 89.85,28.26 IC105.2 | 89.85,30.8 IC105.8 | 89.85,28.26 89.85,30.8 | 89.85,30.8 89.85,35.56 89.22,36.2 IC104.9 85.09,33.97 78.74,33.97 IC201.9 | 95.25,30.8 96.52,30.8 97.47,31.75 97.47,58.74 94.61,61.59 IC103.4 90.81,63.18 89.85,64.14 72.71,64.14 72.39,63.82 | 13.34,24.77 V101.GND | 89.85,16.19 89.85,13.02 87.95,11.18 87.95,9.53 X101.4 87.95,9.21 86.81,8.06 X101.5 | DC201.1 C202.2 72.39,63.5 72.39,63.82 | OK201.5 72.39,63.82
  pour Bottom: 11.11,37.47 20,37.47 20.95,36.51 20.95,17.14 10.79,17.14 10.16,17.78 10.16,36.51
GNDA  (via drill 0.5)
  Top 0.813: IC202.8 83.19,77.47 85.72,74.93 IC202.2 | OK202.5 58.1,72.39 57.15,73.34 57.15,85.09 58.1,86.04 v79.06,86.04 85.09,86.04 86.04,87 CON201.1
  Bottom 0.813: DC201.3 C201.2 65.72,66.04 OK202.5 | IC202.8 83.19,82.87 80.01,86.04 v79.06,86.04
LED-G
  Top 0.406: R106.1 25.72,31.11 IC101.2
LED-R
  Top 0.406: R105.1 30.8,30.8 IC101.4
MISO  (via drill 0.5)
  Top 0.406: IC101.7 v38.42,41.91 37.15,43.18 v37.15,62.23 | v89.22,47.62 89.22,58.1 88.27,59.05 86.36,59.05 85.72,59.69 IC103.2
  Bottom 0.406: IC104.15 92.71,48.9 91.44,47.62 v89.22,47.62 85.41,47.62 IC201.15 80.01,48.9 78.74,47.62 75.25,47.62 69.53,41.91 v38.42,41.91 | SV101.1 v37.15,62.23
MOSI  (via drill 0.5)
  Top 0.406: v91.12,45.09 91.12,58.42 92.08,59.37 92.08,65.72 90.81,66.99 IC103.5 | IC101.6 v35.88,40.96 34.61,42.23 v34.61,66.04
  Bottom 0.406: IC104.14 92.71,46.35 91.44,45.09 v91.12,45.09 85.41,45.09 IC201.14 80.01,46.35 78.74,45.09 75.25,45.09 71.12,40.96 v35.88,40.96 | SV101.4 8.89,66.04 v34.61,66.04
N$1  (via drill 0.5)
  Top 0.406: v92.08,55.24 92.08,32.38 90.49,30.8 IC105.1
  Bottom 0.406: v92.08,55.24 90.81,56.52 IC104.1
N$2  (via drill 0.5)
  Top 0.406: v93.03,52.7 93.03,34.61 93.98,33.66 96.2,33.66 97.47,32.38 97.47,25.4 96.52,24.45 93.66,24.45 92.39,23.18 IC105.4
  Bottom 0.406: v93.03,52.7 91.76,53.98 IC104.2
N$3  (via drill 0.5)
  Top 0.406: v15.24,87 v43.5,87
  Bottom 0.406: LED201.K v15.24,87 | v43.5,87 43.5,77.79 IC203.3
N$5
  Top 0.406: R206.1 21.27,67.31 22.54,68.58 22.54,71.75 26.35,75.56 26.35,78.74 27.3,79.69 Q201.1 28.57,80.64 29.84,81.92 43.81,81.92 44.77,80.96 IC203.2
  Bottom 0.61: JP1.3 29.53,80.64 Q201.1
N$6
  Top 0.813: C105.1 15.24,28.26 15.4,28.1
  Top 1.27: C106.+ 15.88,46.35 14.92,47.31 6.35,47.31 5.71,46.67 5.71,43.81 6.35,43.18 8.89,43.18 9.53,42.55 9.53,30.48 10.16,29.84 D102.C 13.65,29.84 15.4,28.1 V101.IN
N$8  (via drill 0.5)
  Top 0.406: R207.1 24.13,67.31 25.4,68.58 v25.4,73.03
  Top 0.61: IC203.7 32.07,76.52 | 32.07,76.52 Q202.1 | v32.07,80.96 32.07,76.52
  Bottom 0.406: v25.4,73.03 Q202.1
  Bottom 0.61: JP1.4 v32.07,80.96
N$9
  Top 0.406: R105.2 29.84,6.35 28.89,5.4 D101.AR
N$10
  Top 0.406: R201.2 75.25,59.05 76.52,57.78 IC201.1
N$13
  Top 0.406: R106.2 26.99,8.89 26.04,7.94 20.95,7.94 20,6.99 D101.AG
N$40
  Top 0.406: IC202.1 75.88,73.03 75.25,73.66 71.12,73.66 69.53,72.07 R203.1
  Bottom 0.406: OK202.6 60.64,74.93 61.91,73.66 66.99,73.66 69.53,71.12 R203.1
N$43
  Top 0.406: R204.1 61.59,66.36 62.23,66.99 62.23,74.3 62.87,74.93 OK201.3
N$44  (via drill 0.5)
  Top 0.406: R204.2 68.26,66.36 67.31,67.31 67.31,73.66 68.9,75.25 68.9,82.23 69.53,82.87 88.9,82.87 89.53,82.23 89.53,79.06 v90.81,77.79
  Bottom 0.406: v90.81,77.79 IC202.4
N$46
  Top 0.406: OK202.3 53.34,74.93 54.29,73.98 54.29,67.63 57.47,64.45 73.66,64.45 75.25,66.04 R201.1
N$48  (via drill 0.5)
  Top 0.406: v80.33,66.04 80.33,55.56 78.74,53.98 IC201.2
  Bottom 0.406: OK201.6 73.98,74.93 78.11,70.8 R202.1 78.11,68.26 v80.33,66.04
PLUGGED  (via drill 0.5)
  Top 0.406: IC101.39 25.72,36.51 26.99,35.24 26.99,32.38 28.57,30.8 v28.57,18.1 | CON101.3 14.53,12.62 16.19,14.29 19.68,14.29 23.5,18.1 v25.08,18.1
  Bottom 0.406: v25.08,18.1 v28.57,18.1
Q-CLK  (via drill 0.5)
  Top 0.813: QG101.8 v73.98,38.73
  Bottom 0.813: IC101.13 53.66,32.38 54.61,31.43 65.09,31.43 67.63,28.89 QG101.8 | IC104.8 86.04,40.01 81.28,40.01 80.01,38.73 IC201.8 v73.98,38.73
RXD-TTL  (via drill 0.5)
  Top 0.406: IC101.14 v56.2,36.83 | v24.45,36.83 24.45,55.88 22.86,57.47 18.73,57.47 R208.1 | Q201.3 28.26,77.15 27.3,76.2 v27.3,59.37
  Bottom 0.406: v56.2,36.83 v24.45,36.83 | v27.3,59.37 16.83,59.37 R208.1
SCK  (via drill 0.5)
  Top 0.406: IC101.8 v40.96,40.01 40.96,41.91 39.69,43.18 v39.69,64.77 | v90.17,42.55 90.17,59.05 89.53,59.69 89.53,65.72 88.27,66.99 IC103.6
  Bottom 0.406: IC104.13 92.71,43.81 91.44,42.55 v90.17,42.55 85.41,42.55 IC201.13 80.01,43.81 78.74,42.55 74.61,42.55 72.07,40.01 v40.96,40.01 | SV101.3 v39.69,64.77
SCL  (via drill 0.5)
  Top 0.406: IC101.22 v68.9,44.77 | v60.01,62.23 v60.01,44.77 52.39,37.15 52.39,31.75 52.07,31.43 R108.1
  Bottom 0.406: v68.9,44.77 v60.01,44.77 | v60.01,62.23 JP202.3
SDA  (via drill 0.5)
  Top 0.406: v57.47,46.67 57.47,62.55 55.24,64.77 JP202.4 | R107.1 49.21,31.43 49.85,32.07 49.85,41.59 51.44,43.18 v51.44,46.67
  Bottom 0.406: IC101.23 66.36,46.99 66.04,46.67 v57.47,46.67 v51.44,46.67
SPG  (via drill 0.5)
  Top 0.406: v23.18,53.98 IC101.40
  Bottom 0.406: R109.2 20.32,53.98 v23.18,53.98 30.48,53.98 R110.1
TXD-TTL  (via drill 0.5)
  Top 0.406: IC101.15 v58.74,37.78 | v26.99,37.78 26.99,54.93 | 26.99,54.93 23.5,58.42 20.64,58.42 R209.1 | Q202.3 28.57,56.52 26.99,54.93
  Bottom 0.406: v58.74,37.78 v26.99,37.78
V-NETZTEIL
  Bottom 1.27: D103.A 6.67,24.13 8.26,22.54 8.26,14.92 CON101.1
(copper drawn outside any net)
  shapes: Bottom area x1

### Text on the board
Bottom: MBCAN-Projekt | 01-10-2021 | (c) Dr.-Ing. Th. Wiesner | mbc80.brd | bottom
tNames: PIN 6 - ohne Funktion | PIN 5 - CAN Low | + | FTDI 3V3 | PIN 4 - ohne Funktion | PIN 3 - CAN High | PIN 2 - ohne Funktion | CONNECT | PIN 1 - Masse | GND | RxD | TxD | *) siehe BD | SDA | SCL | +5V | STATUS | MBCAN-Projekt | DC | (c) Dr.-Ing. Th. Wiesner | OUT | HW: 21.10.01 | +18V | mbc-80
